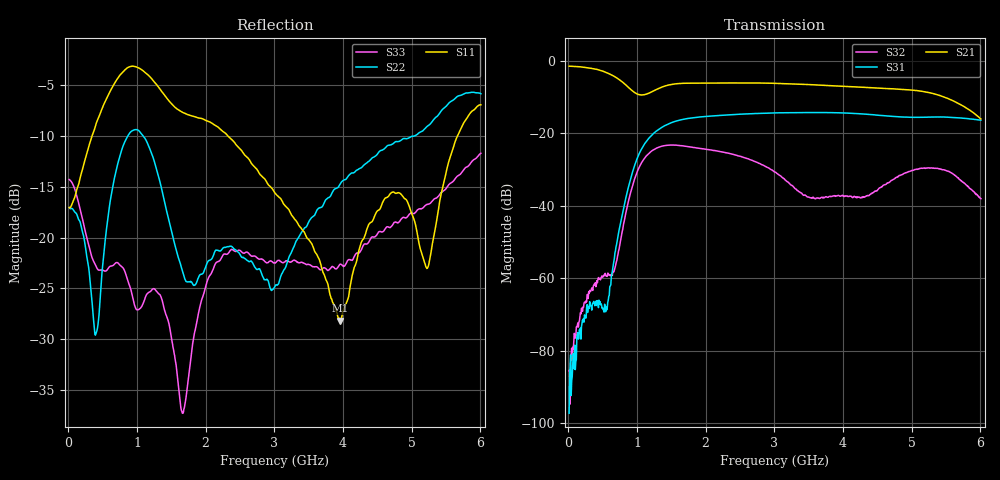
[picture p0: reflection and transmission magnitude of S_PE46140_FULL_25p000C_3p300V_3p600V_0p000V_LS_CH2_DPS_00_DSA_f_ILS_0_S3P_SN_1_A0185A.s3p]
! Device ID: PE46140_FULL
! File Path: z:\PE46140\MajorStates\25p000C\3p300\LS_CH2_DPS_00_DSA_f_ILS_0\PE46140_FULL_25p000C_3p300V_3p600V_0p000V_LS_CH2_DPS_00_DSA_f_ILS_0_S3P_SN_1_A0185A.s3p
! Serial: 1
! Lot: A0185A
! Temp: 25.000C
! VDD: 3.300
! VSS: 0.000
! Control_Hi: 3.600
! Control_Lo: 0.000
! Logic State: LS_CH2_DPS_00_DSA_f_ILS_0
! Port 1: RFIN
! Port 2: RFOUT1
! Port 3: RFOUT2
! ThroughPath:1-3
! IDD: 0.0003147637
! ISS: -1.395e-007
! Comment:
#  Hz  S  RI  R  50
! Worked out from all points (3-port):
!   801 points, 10 MHz to 6.01 GHz, reference 50 ohm
!   strongest paths, dB at 10 MHz, 1.51 GHz, 3.01 GHz, 4.51 GHz, 6.01 GHz:
!     S21: -1.5, -6.5, -6.2, -7.6, -16.1
!     S31: -97.2, -17.0, -14.4, -15.0, -16.4
!     S32: -85.5, -23.2, -30.7, -35.5, -38.0
!   lowest |S11| = -28.2 dB at 3.962 GHz (marker M1), VSWR 1.08, Z = 47.1 + j2.45 ohm
!   |S11| at or under -10 dB: start of sweep to 346.1 MHz; 2.318 GHz to 5.672 GHz (3.353 GHz wide, 83.9 % of centre)
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1e7  0.1401 -0.0109  0.8421 -0.0244  8.88e-06 4.56e-07
     0.8419 -0.0243  0.1399 -0.00679  -5.59e-05 -1.91e-05
     -1.18e-05 7.04e-06  2.21e-06 5.28e-05  0.1918 -0.0163
4e8  -0.0601 -0.3534  0.3772 -0.6607  -0.000502 -9.33e-05
     0.3801 -0.6642  -0.0277 -0.0191  -6.72e-05 0.000806
     -0.000479 -5.74e-05  1.91e-05 0.000767  -0.0713 -0.0134
5.65e8  -0.2683 -0.4072  0.0521 -0.6778  7.68e-05 0.000426
        0.0525 -0.678  -0.0215 0.1153  0.0007 0.000855
        -4.85e-05 0.000384  0.000672 0.000825  -0.0413 0.0558
1.18e9  -0.5727 0.2329  -0.211 -0.2908  -0.0868 -0.00341
        -0.2111 -0.2913  0.198 -0.191  0.00524 0.0535
        -0.087 -0.00334  0.00511 0.0536  0.0479 0.0247
1.6675e9  -0.287 0.2929  -0.4867 -0.0383  0.0983 0.1199
          -0.4869 -0.0388  0.0332 -0.059  0.00123 -0.0669
          0.0983 0.1203  0.00141 -0.067  0.0136 0.00171
3.01e9  0.0503 0.1573  0.4045 0.2744  -0.168 -0.09
        0.4043 0.2752  -0.0575 -0.00204  0.0264 -0.0119
        -0.1684 -0.0901  0.0267 -0.012  0.0675 0.0324
3.9625e9  -0.0293 0.0259  0.1084 -0.4327  -0.0241 0.1896
          0.1089 -0.4329  0.1273 0.1329  0.00605 0.0122
          -0.0237 0.1898  0.00612 0.0121  0.0624 0.0396
4.8025e9  -0.1655 -0.0123  -0.4062 -0.014  0.1675 0.0235
          -0.4065 -0.0147  0.2941 0.0257  -0.0252 -0.00112
          0.1674 0.023  -0.025 -0.000896  0.1177 0.00793
5.23e9  -0.0478 -0.052  -0.1972 0.3099  0.139 -0.0924
        -0.1981 0.3096  0.3513 -0.0141  -0.00524 0.033
        0.1391 -0.0923  -0.00525 0.0327  0.1442 0.0175
6.01e9  -0.3505 -0.2787  0.1506 0.0446  -0.0723 -0.1325
        0.1508 0.0447  0.2473 -0.4431  0.0119 -0.00343
        -0.073 -0.1328  0.0121 -0.0034  0.2561 0.038
